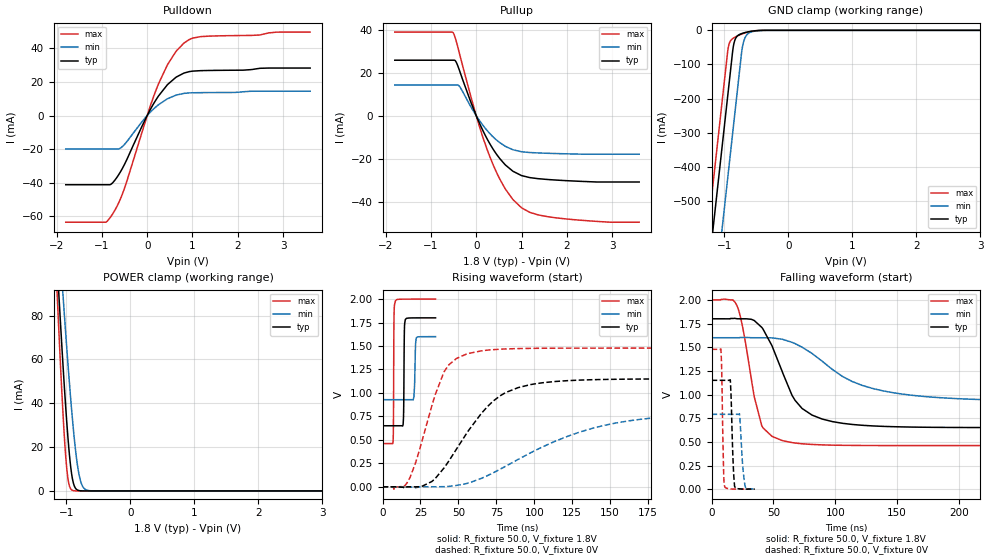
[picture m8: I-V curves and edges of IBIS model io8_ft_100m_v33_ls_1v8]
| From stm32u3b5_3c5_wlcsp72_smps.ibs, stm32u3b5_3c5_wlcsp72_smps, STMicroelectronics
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[Model]   io8_ft_100m_v33_ls_1v8
Model_type I/O
Polarity   Non-Inverting
Enable   Active-Low
| CAP_THRESHOLD on pad IOFT is "UDTCAPC" :
| Rising=30.0% of vddiom   Falling=70.0% of vddiom
| C_comp min and max val. don't necessarily correlate with the min and max pvt
| but are the smallest and greatest pad capacitance found.
| var   typ   min   max
C_comp   4.46110pF  4.37696pF  4.58318pF
|C_comp_pullup   2.75008pF  2.57391pF  2.90899pF
|C_comp_pulldown   1.71102pF  1.80306pF  1.67419pF
Vinl = 800.0mV
Vinh = 1.0V
Vmeas = 900.0mV   | Reference voltage for timing measurements
Cref  = 50.0pF   | Timing specification test load capacitance value
Rref  = 1.0MOhm   | Timing specification test load resistance value
Vref  = 990.0mV   | Timing specification test load voltage
[Model Spec]
| TIME_THRESHOLD on pin ZIV33M is "CMOS" :
| Rising=50.0% of vddiom   Falling=50.0% of vddiom
Vinl 689.50000mV 614.50000mV 772.50000mV
Vinh 1.08250V 955.50000mV 1.18750V
| variable   typ   min   max
[Temperature Range] 25.0 130.0 -40.0
| variable   typ   min   max
[Voltage Range] 1.8V 1.6V 2.0V
| variable   typ   min   max
[POWER Clamp Reference] 1.8V 1.6V 2.0V
| variable   typ   min   max
[GND Clamp Reference] 0V 0V 0V
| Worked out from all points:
|   slope of the pulldown table from 0 to 0.27 V, typ, clamps not added: 21.9 ohm
|   slope of the pullup table from 0 to 0.27 V, typ, clamps not added: 22.7 ohm
|   GND clamp passes 1 mA (typ) near -0.50 V on its own axis
|   POWER clamp passes 1 mA (typ) near -0.85 V on its own axis
|   rising waveform, R_fixture 50.0, V_fixture 1.8V: 20-80 % time 339ps typ, 621ps min, 266ps max; typ from 0.65 V to 1.8 V
|   falling waveform, R_fixture 50.0, V_fixture 1.8V: 20-80 % time 24.7ns typ, 53.2ns min, 13.2ns max; typ from 1.8 V to 0.65 V
|   rising waveform, R_fixture 50.0, V_fixture 0V: 20-80 % time 31.7ns typ, 66.7ns min, 17ns max; typ from 0 V to 1.15 V
|   falling waveform, R_fixture 50.0, V_fixture 0V: 20-80 % time 1.69ns typ, 2.37ns min, 1.26ns max; typ from 1.15 V to 0 V
[POWER Clamp]
-1.8V     478.8mA    439.5mA    561.1mA
-1.14V    101.7mA    127.5mA    87.74mA
-1.11V    86.11mA    114.3mA    68.77mA
-1.05V    56.42mA    88.49mA    34.19mA
-1.01V    38.33mA    71.95mA    15.91mA
-970mV    22.56mA    56.16mA    4.74mA
-910mV    6.426mA    34.56mA    354.8uA
-850mV    950.4uA    17.03mA    20.6uA
-800mV    153.4uA    7.248mA    1.891uA
-750mV    23.75uA    2.361mA    173.6nA
-670mV    1.188uA    286.7uA    3.927nA
3.6V      0A         0A         0A
[GND Clamp]
-1.8V     -1.641A    -1.882A    -1.509A
-1.24V    -689.3mA   -929.9mA   -557.3mA
-1.05V    -366.3mA   -606.9mA   -234.3mA
-950mV    -196.3mA   -436.9mA   -64.35mA
-930mV    -162.3mA   -402.9mA   -42.64mA
-870mV    -60.33mA   -300.9mA   -24.14mA
-850mV    -37.9mA    -266.9mA   -21.7mA
-770mV    -12.83mA   -130.9mA   -14.29mA
-730mV    -9.517mA   -63.9mA    -11.18mA
-690mV    -7.204mA   -27.69mA   -8.428mA
-530mV    -1.58mA    -2.534mA   -1.415mA
3.6V      1.308nA    187.1nA    582.2pA
| variable   typ   min   max
[Pullup Reference] 1.8V 1.6V 2.0V
| variable   typ   min   max
[Pulldown Reference] 0V 0V 0V
[Pullup]
-1.8V     25.79mA    14.24mA    38.86mA
-510mV    25.79mA    14.24mA    38.56mA
-450mV    25.15mA    14.24mA    35.19mA
-370mV    20.99mA    13.61mA    28.84mA
20mV      -1.001mA   -644.5uA   -1.446mA
300mV     -13.02mA   -8.285mA   -19mA
460mV     -18.26mA   -11.51mA   -26.87mA
650mV     -23mA      -14.3mA    -34.27mA
1V        -27.82mA   -16.74mA   -42.77mA
1.37V     -29.26mA   -17.3mA    -46.1mA
1.74V     -29.87mA   -17.57mA   -47.39mA
3.6V      -30.8mA    -17.88mA   -49.48mA
[Pulldown]
-1.8V     -41.16mA   -19.96mA   -63.43mA
-920mV    -41.16mA   -19.96mA   -63.43mA
-780mV    -40.43mA   -19.96mA   -59.18mA
-620mV    -34.74mA   -19.77mA   -51.3mA
-510mV    -29.46mA   -17.38mA   -43.8mA
0V        155.1fA    35.29pA    0A
250mV     11.64mA    6.428mA    18.87mA
460mV     18.67mA    10.12mA    30.76mA
630mV     22.61mA    12.05mA    37.86mA
810mV     25.21mA    13.14mA    43.03mA
1.18V     26.67mA    13.59mA    46.9mA
3.6V      28.21mA    14.43mA    49.6mA
[Ramp]
dV/dt_r 690.00845mV/31.61644ns 474.1583mV/66.47645ns 886.3634mV/16.63672ns
dV/dt_f 689.75442mV/24.13751ns 402.76082mV/52.87637ns 923.68047mV/12.21755ns
R_load = 50.0
| Removed startup time: 0s 0s 0s  .
| Removed end time: 34.95ns.
[Rising Waveform]
R_fixture   = 50.0
V_fixture   = 1.8V
V_fixture_min = 1.6V
V_fixture_max = 2.0V
0s        650.4mV    928.3mV    460.5mV
6.9ns     650.4mV    928.3mV    477.5mV
7.2ns     650.4mV    928.3mV    728.3mV
7.55ns    650.4mV    928.3mV    1.801V
8.55ns    650.4mV    928.3mV    1.983V
13.55ns   663.2mV    928.3mV    1.999V
15ns      1.782V     928.3mV    1.999V
20.7ns    1.799V     961.6mV    1.999V
22.15ns   1.799V     1.583V     1.999V
34.95ns   1.799V     1.6V       2V
| Removed startup time: 0s 0s 0s  .
| Removed end time: 397.95ns.
[Falling Waveform]
R_fixture   = 50.0
V_fixture   = 1.8V
V_fixture_min = 1.6V
V_fixture_max = 2.0V
0s        1.8V       1.6V       2V
19.75ns   1.802V     1.6V       1.959V
24.35ns   1.8V       1.603V     1.76V
34.45ns   1.782V     1.6V       977.6mV
40.6ns    1.709V     1.6V       668.3mV
56.85ns   1.251V     1.585V     514.6mV
73.1ns    852.8mV    1.5V       479.6mV
105.6ns   696.3mV    1.192V     463.5mV
178.7ns   653.5mV    971.8mV    460.6mV
398ns     650.4mV    928.7mV    460.5mV
| Removed startup time: 0s 0s 0s  .
| Removed end time: 397.9ns.
[Rising Waveform]
R_fixture   = 50.0
V_fixture   = 0V
V_fixture_min = 0V
V_fixture_max = 0V
0s        5.001nV    122.3nV    3.682nV
16.25ns   -371.6uV   598.7nV    44.97mV
21.95ns   -192.9uV   -9.839mV   264.6mV
32.5ns    56.43mV    -57.57uV   863.9mV
40.6ns    202.4mV    1.747mV    1.227V
56.85ns   603.7mV    41.16mV    1.421V
73.1ns    915.7mV    150.6mV    1.461V
89.35ns   1.056V     291.8mV    1.472V
162.5ns   1.147V     702.9mV    1.477V
397.9ns   1.15V      790.3mV    1.477V
| Removed startup time: 0s 0s 0s  .
| Removed end time: 34.95ns.
[Falling Waveform]
R_fixture   = 50.0
V_fixture   = 0V
V_fixture_min = 0V
V_fixture_max = 0V
0s        1.15V      790.6mV    1.477V
7.5ns     1.15V      790.6mV    1.479V
8.15ns    1.15V      790.6mV    1.267V
9.75ns    1.15V      790.6mV    184.2mV
10.7ns    1.15V      790.6mV    22.49mV
15.15ns   1.149V     790.6mV    3.156mV
18.55ns   33.28mV    790.6mV    1.268mV
22.6ns    3.522mV    791.1mV    620.4uV
27.15ns   1.062mV    28.34mV    307.5uV
34.95ns   494.2uV    2.7mV      151uV
